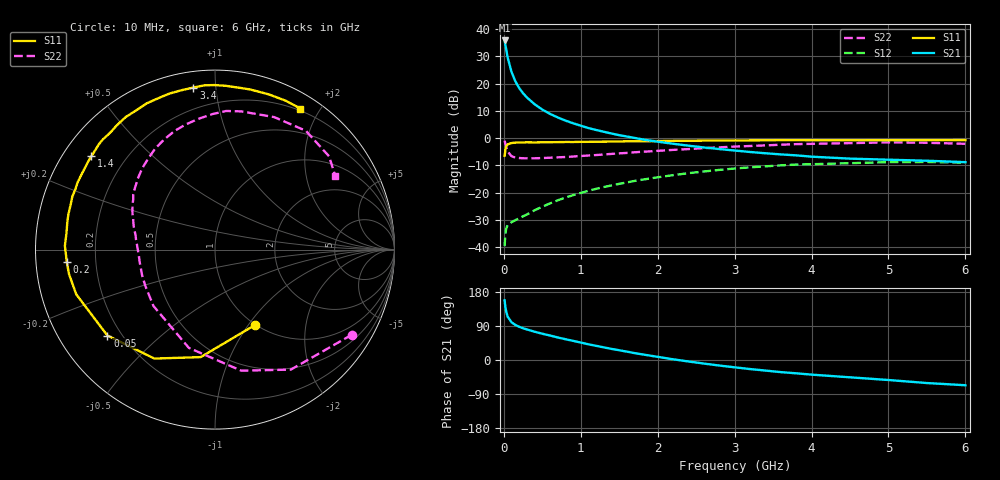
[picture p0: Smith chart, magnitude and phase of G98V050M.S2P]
! SIEMENS Small Signal Semiconductors
! BFG235
! Si NPN RF Bipolar Junction Transistor in SOT223
! VCE = 8 V  IC = 50 mA
! Common Emitter S-Parameters:  July  1994
# GHz  S  MA  R  50
!  f  S11  S21  S12  S22
! GHz  MAG  ANG  MAG  ANG  MAG  ANG  MAG  ANG
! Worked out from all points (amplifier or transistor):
!   40 points, 10 MHz to 6 GHz, reference 50 ohm
!   highest |S21| = 35.8 dB at 10 MHz (marker M1)
!   |S21| within 3 dB of that: start of sweep to 28.87 MHz
!   unconditionally stable (mu >= 1): 529.6 MHz to 1.316 GHz
!   at 200 MHz: K = 0.66, MSG = 23.9 dB, |S12| = -29.4 dB
!   at 1.5 GHz: K = 0.98, MSG = 8.9 dB, |S12| = -16.8 dB
!   at 6 GHz: K = 0.91, MSG = 0.1 dB, |S12| = -9.0 dB
!   S11 on the Smith chart (normalised r, x): 10 MHz: 0.99, -1.08; 50 MHz: 0.15, -0.34; 200 MHz: 0.09, -0.04; 1.4 GHz: 0.08, +0.33; 3.4 GHz: 0.08, +0.87; 6 GHz: 0.17, +1.76
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0.01  0.4756 -62.0  61.82 157.6  0.0104 70.0  0.8977 -31.9
0.02  0.6044 -97.6  51.78 140.5  0.0174 55.0  0.7911 -57.7
0.03  0.6947 -119.1  42.84 128.3  0.0215 44.9  0.6901 -77.8
0.05  0.7672 -141.4  29.88 114.2  0.0255 34.7  0.5666 -104.9
0.1  0.8121 -162.1  16.25 99.5  0.0286 30.2  0.465 -137.5
0.15  0.8246 -170.4  10.99 92.4  0.0312 33.2  0.438 -152.2
0.2  0.8286 -175.1  8.243 87.6  0.0339 36.8  0.4307 -160.5
0.25  0.8319 -178.8  6.645 83.8  0.0368 40.2  0.426 -165.9
0.3  0.8366 178.5  5.554 80.6  0.0397 43.6  0.4255 -170.2
0.4  0.8327 173.4  4.175 74.6  0.0474 47.7  0.4258 -175.9
0.5  0.8371 169.3  3.336 69.3  0.055 50.5  0.4306 179.8
0.6  0.8402 166.4  2.781 64.6  0.0633 52.1  0.4363 176.0
0.7  0.8425 162.6  2.394 59.5  0.072 53.0  0.4434 172.8
0.9  0.8472 156.9  1.871 50.5  0.0897 52.4  0.4586 167.2
1.1  0.8537 150.3  1.527 41.3  0.1079 50.9  0.479 161.7
1.4  0.8631 142.9  1.212 29.3  0.1355 46.8  0.5128 153.8
2.2  0.8903 124.0  0.787 1.9  0.2088 31.3  0.6077 131.9
3.2  0.9073 102.0  0.556 -23.9  0.2903 7.6  0.7157 103.3
3.4  0.911 97.6  0.527 -27.9  0.3031 2.6  0.7347 97.1
4.5  0.9136 77.7  0.42 -45.7  0.3465 -23.7  0.8086 65.9
5.5  0.9183 64.5  0.384 -60.8  0.3645 -46.3  0.821 39.3
6  0.9187 58.8  0.362 -66.6  0.353 -54.7  0.7853 31.4
